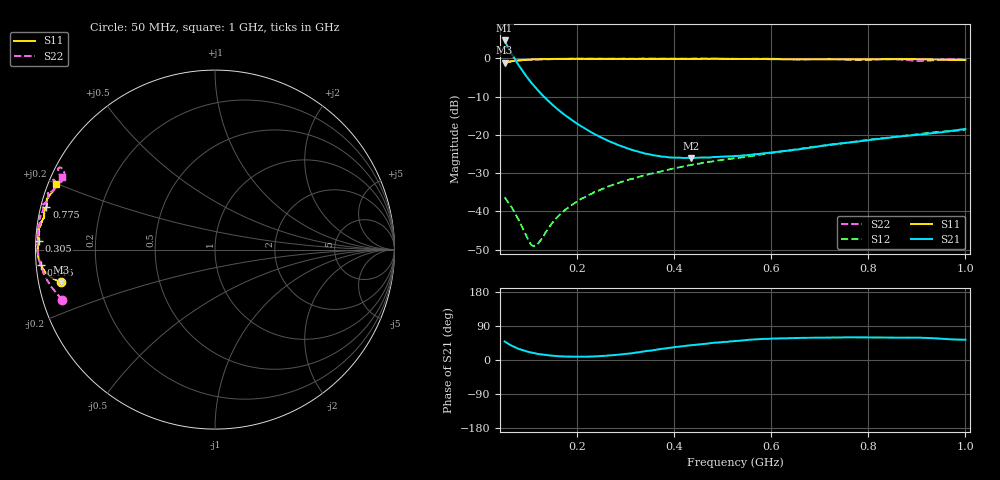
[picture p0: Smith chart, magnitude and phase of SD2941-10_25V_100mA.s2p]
!Agilent Technologies,E8358A,US42080673,A.04.86
!Agilent E8358A: A.04.86
!Date: Friday, June 09, 2006 14:43:23
!Correction: S11(Full 2 Port SOLT,1,2) S21(Full 2 Port SOLT,1,2) S12(Full 2 Port SOLT,1,2) S22(Full 2 Port SOLT,1,2)
!S2P File: Measurements: S11, S21, S12, S22:
# Hz S  MA  R 50
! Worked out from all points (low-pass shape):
!   191 points, 50 MHz to 1 GHz, reference 50 ohm
!   highest |S21| = 4.70 dB at 50 MHz (marker M1); lowest = -26.1 dB at 435 MHz (marker M2)
!   |S21| within 3 dB of the highest: start of sweep to 62.46 MHz
!   lowest |S11| = -1.2 dB at 50 MHz (marker M3), VSWR 15.09, Z = 3.35 - j5.23 ohm
!   |S11| at or under -10 dB: nowhere
!   |S22| runs from -1.0 to 0.0 dB; largest |S21 - S12| = 1.7
!   S11 on the Smith chart (normalised r, x): 50 MHz: 0.07, -0.10; 115 MHz: 0.01, -0.04; 305 MHz: 0.01, +0.02; 775 MHz: 0.02, +0.13; 1 GHz: 0.02, +0.20
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5e7  0.8757 -168.0  1.717 48.9  0.01525 -29.9  0.8954 -161.7
5.5e7  0.893 -168.7  1.479 44.9  0.01373 -32.3  0.9045 -163.0
6e7  0.9058 -169.3  1.295 40.9  0.01242 -34.1  0.9134 -164.3
6.5e7  0.9173 -169.9  1.138 37.3  0.01118 -35.1  0.9214 -165.4
7.5e7  0.9355 -171.1  0.8909 31.6  0.008584 -34.5  0.9355 -167.2
9e7  0.9568 -172.7  0.6426 24.7  0.005569 -25.9  0.9503 -169.6
1.05e8  0.9663 -174.2  0.4812 19.7  0.003628 1.8  0.96 -171.7
1.15e8  0.9734 -174.9  0.4053 17.2  0.003594 28.2  0.9664 -172.9
1.6e8  0.9845 -177.7  0.2146 10.1  0.008575 75.7  0.9831 -176.8
2.1e8  0.9887 -179.6  0.1271 8.8  0.01486 80.7  0.9892 -180.0
2.65e8  0.9865 178.4  0.08276 12.1  0.02126 80.8  0.9878 177.3
3.05e8  0.9824 177.3  0.06606 16.7  0.02584 80.1  0.9906 175.4
3.7e8  0.9876 176.0  0.05247 28.6  0.03296 79.1  0.9903 172.9
4.35e8  0.9838 174.1  0.04974 39.1  0.0404 76.4  0.9919 170.2
5.25e8  0.9849 172.4  0.05292 50.1  0.04946 73.4  0.9807 167.6
6.85e8  0.9737 168.4  0.06879 58.6  0.06951 69.6  0.9767 162.0
7.75e8  0.9697 165.7  0.08131 59.9  0.08196 66.8  0.9543 159.1
8.45e8  0.9764 163.9  0.09213 58.9  0.09243 64.8  0.9804 156.7
8.95e8  0.9764 162.6  0.09911 58.8  0.1009 63.0  0.936 156.2
9.3e8  0.9665 161.3  0.105 58.0  0.107 62.1  0.9397 153.2
9.6e8  0.9608 159.8  0.1104 55.2  0.111 60.5  0.9787 152.1
1e9  0.9578 157.6  0.1195 53.6  0.117 56.9  0.9453 154.6
